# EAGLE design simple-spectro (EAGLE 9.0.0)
DELETE: MF
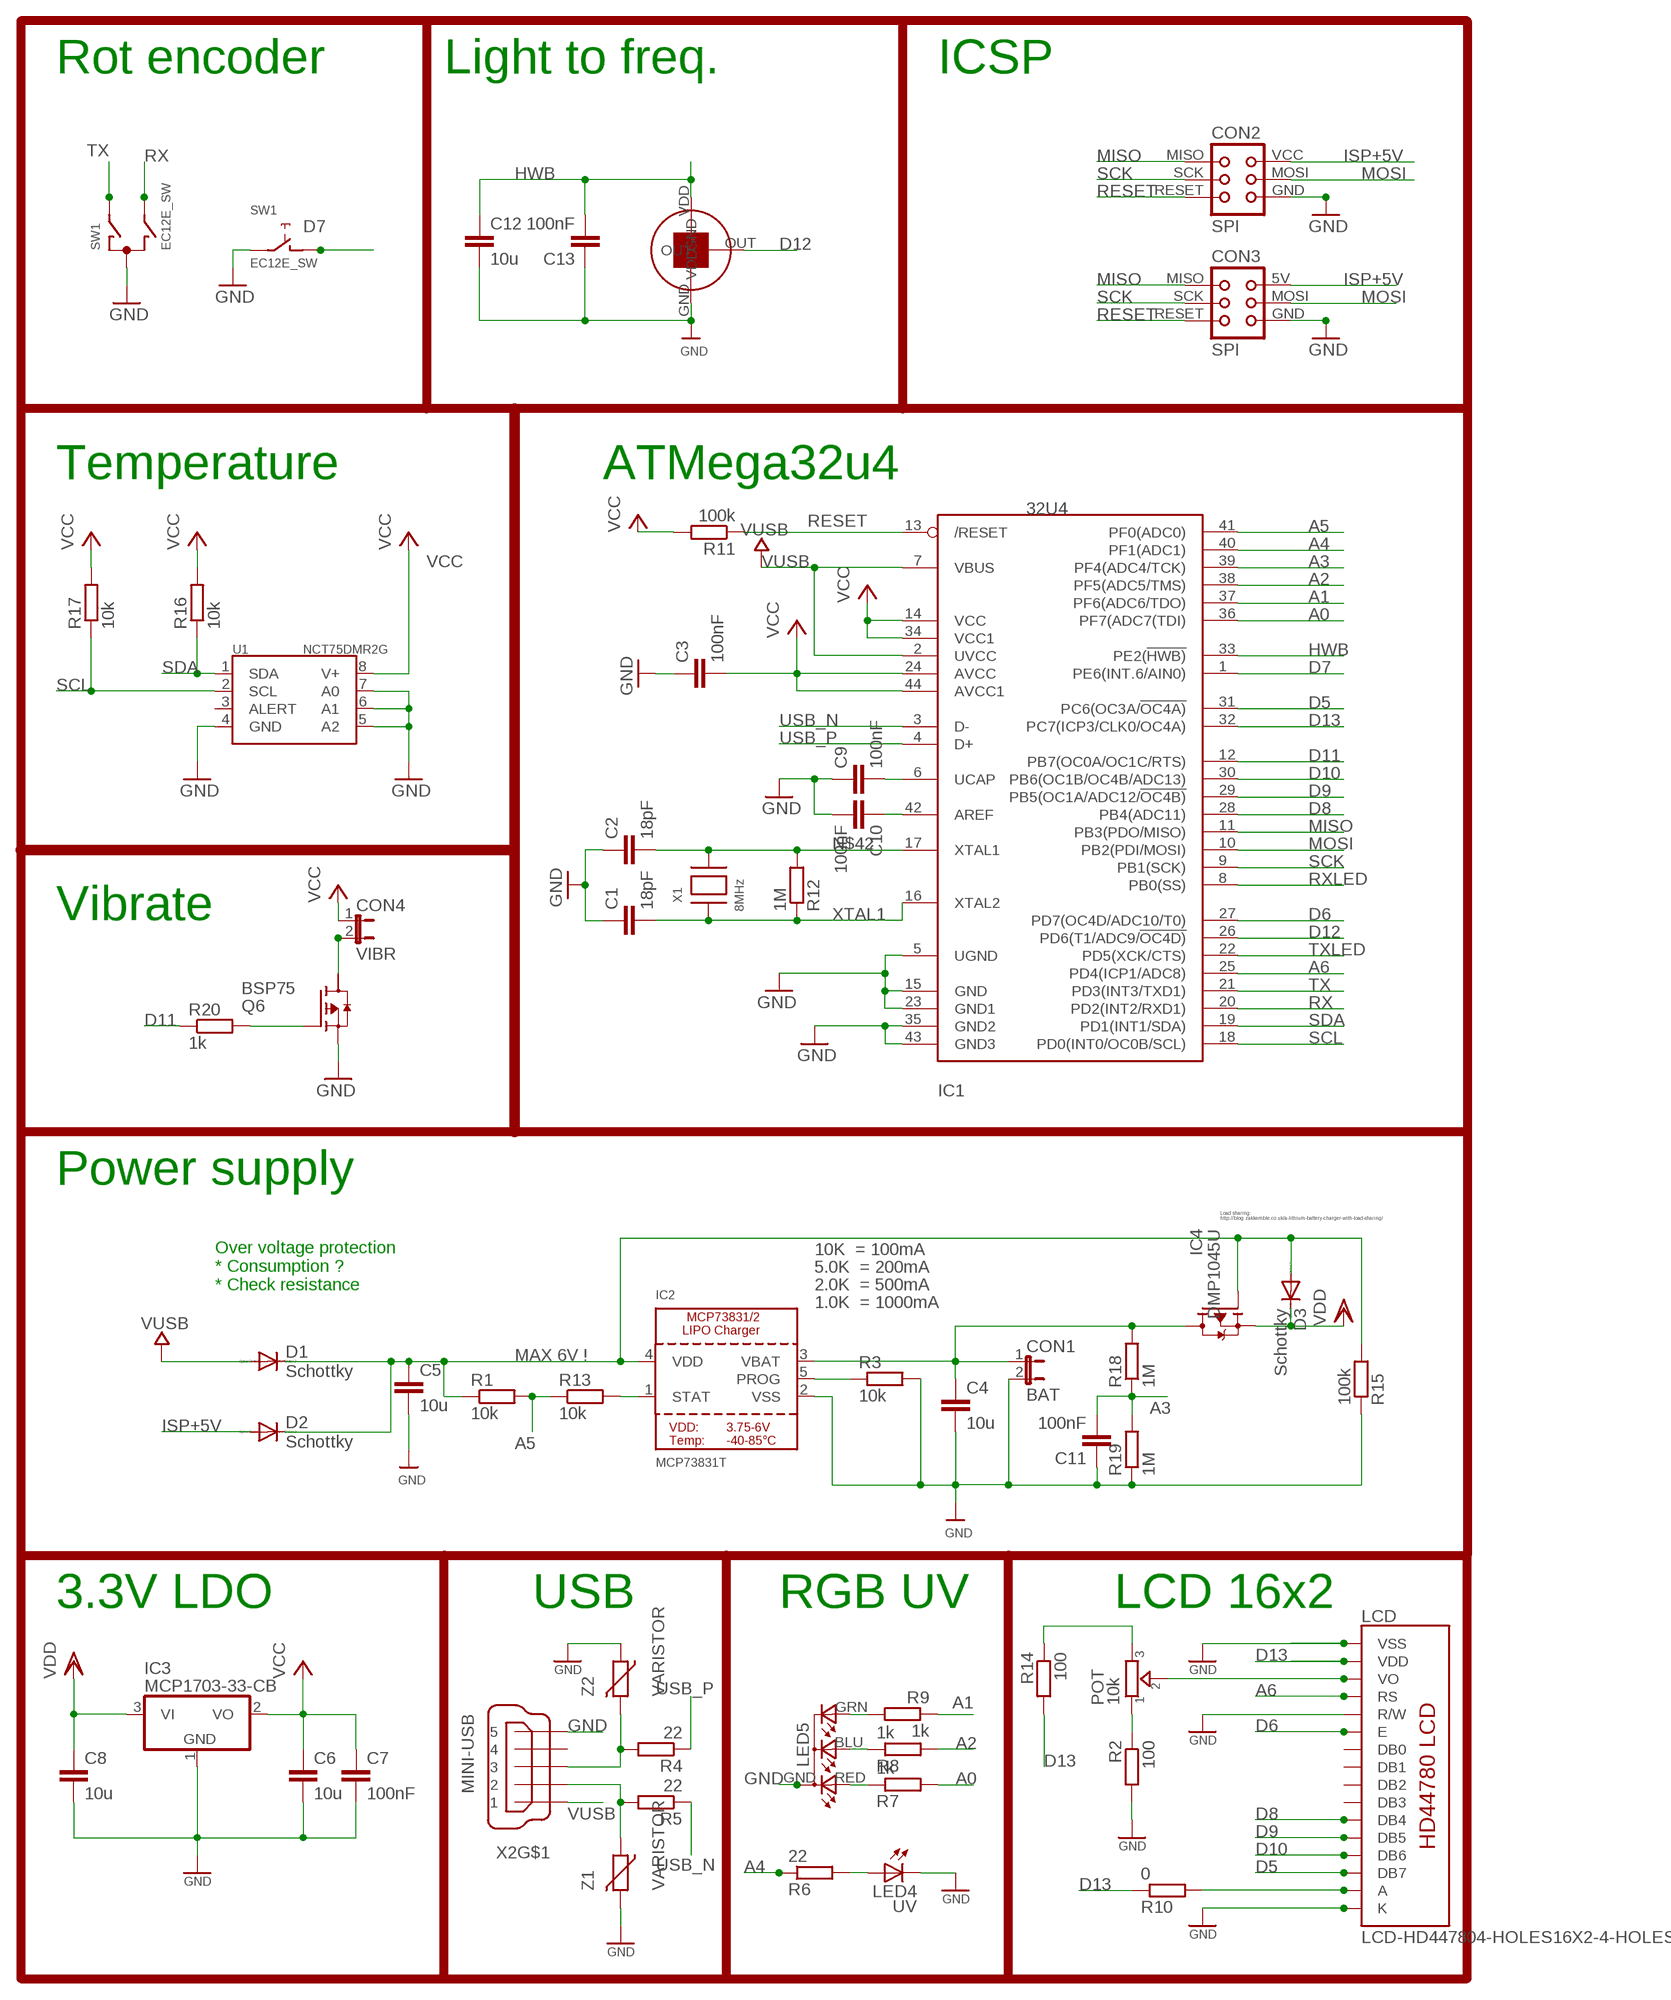
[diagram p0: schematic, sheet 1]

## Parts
C1  18pF  C-EUC0805K  [C0805K]
C2  18pF  C-EUC0805K  [C0805K]
C3  100nF  C-EUC0805K  [C0805K]
C4  10u  C-EUC0805K  [C0805K]
C5  10u  C-EUC0805K  [C0805K]
C6  10u  C-EUC0805K  [C0805K]
C7  100nF  C-EUC0805K  [C0805K]
C8  10u  C-EUC0805K  [C0805K]
C9  100nF  C-EUC0805K  [C0805K]
C10  100nF  C-EUC0805K  [C0805K]
C11  100nF  C-EUC0805K  [C0805K]
C12  10u  C-EUC0805K  [C0805K]
C13  100nF  C-EUC0805K  [C0805K]
CON1  BAT  JP1E  [JP1]
CON2  SPI  TINYISP  [TINYISP]
CON3  SPI  TINYISPT  [TC2030-MCP-NL]
CON4  VIBR  JP1E  [JP1]
D1  Schottky  MBR0520LT  [SOD123]
D2  Schottky  MBR0520LT  [SOD123]
D3  Schottky  MBR0520LT  [SOD123]
IC1  32U4  ATMEGA32U4-AU  [TQFP44]
IC2  MCP73831T  MCP73831/2  [SOT23-5]
IC3  MCP1703-33-CB  MCP1703CB  [SOT23]
IC4  DMP1045U  TRANSISTOR_FET_TSM2301CX  [SOT-23]
LCD  LCD-HD447804-HOLES16X2-4-HOLES  [LCD-16X2-4HOLES]
LED4  UV  LED5MM  [LED5MM]
LED5  RGB-COMMON-CATHODE  [LED-TRICOLOR-THROUGHHOLE]
POT  10k  TRIMMER-3362P  [TRIMMER_3362P]
Q6  BSP75  [PG-SOT-223]
R1  10k  R-EU_R0805  [R0805]
R2  100  R-EU_R0805  [R0805]
R3  10k  R-EU_R0805  [R0805]
R4  22  R-EU_R0805  [R0805]
R5  22  R-EU_R0805  [R0805]
R6  22  R-EU_R0805  [R0805]
R7  1k  R-EU_R0805  [R0805]
R8  1k  R-EU_R0805  [R0805]
R9  1k  R-EU_R0805  [R0805]
R10  0  R-EU_R0805  [R0805]
R11  100k  R-EU_R0805  [R0805]
R12  1M  R-EU_R0805  [R0805]
R13  10k  R-EU_R0805  [R0805]
R14  100  R-EU_R0805  [R0805]
R15  100k  R-EU_R0805  [R0805]
R16  10k  R-EU_R0805  [R0805]
R17  10k  R-EU_R0805  [R0805]
R18  1M  R-EU_R0805  [R0805]
R19  1M  R-EU_R0805  [R0805]
R20  1k  R-EU_R0805  [R0805]
SW1  EC12E_SW  [ALPS_EC12E_SW]
U1  NCT75DMR2G  TMP75DGK  [MSOP8]
U$7  TSL237  [TSL237]
X1  8MHz  XTALNX6035  [NX6035]
X2  MINI-USB  MINI-USB-SCHIELD-32005-201  [32005-201]
Z1  VARISTOR  VARISTORCN0603  [CT/CN0603]
Z2  VARISTOR  VARISTORCN0603  [CT/CN0603]

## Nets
A0: IC1.36(PF7(ADC7(TDI)) R7.2
A1: IC1.37(PF6(ADC6/TDO)) R9.1
A2: IC1.38(PF5(ADC5/TMS)) R8.2
A3: C11.2 IC1.39(PF4(ADC4/TCK)) R18.1 R19.2
A4: IC1.40(PF1(ADC1)) R6.1
A5: IC1.41(PF0(ADC0)) R1.2 R13.1
A6: IC1.25(PD4(ICP1/ADC8)) LCD.4(RS)
AREF: C10.1 IC1.42(AREF)
D5: IC1.31(PC6(OC3A/!OC4A)) LCD.14(DB7)
D6: IC1.27(PD7(OC4D/ADC10/T0)) LCD.6(E)
D7: IC1.1(PE6(INT.6/AIN0)) SW1.D
D8: IC1.28(PB4(ADC11)) LCD.11(DB4)
D9: IC1.29(PB5(OC1A/ADC12/!OC4B)) LCD.12(DB5)
D10: IC1.30(PB6(OC1B/OC4B/ADC13)) LCD.13(DB6)
D11: IC1.12(PB7(OC0A/OC1C/RTS)) R20.1
D12: IC1.26(PD6(T1/ADC9/!OC4D)) U$7.OUT
D13: IC1.32(PC7(ICP3/CLK0/OC4A)) LCD.2(VDD) R10.1 R14.2
GND [power]: C1.1 C2.1 C3.1 C4.2 C5.2 C6.2 C7.2 C8.2 C9.1 C10.2 C11.1 C12.2 C13.1 CON1.2 CON2.GND CON3.GND IC1.5(UGND) IC1.15(GND) IC1.23(GND1) IC1.35(GND2) IC1.43(GND3) IC2.2(VSS) IC3.1(GND) LCD.1(VSS) LCD.5(R/W) LCD.16(K) LED4.K(C) LED5.GND(A2) Q6.3(S) R2.2 R3.2 R15.1 R19.1 SW1.C SW1.E U1.4(GND) U1.5(A2) U1.6(A1) U1.7(A0) U$7.GND X2.5 Z1.2 Z2.1
HWB: C12.1 C13.2 IC1.33(PE2(!HWB)) U$7.VDD
ISP+5V: CON2.VCC CON3.5V(VCC) D2.A
MISO: CON2.MISO CON3.MISO IC1.11(PB3(PDO/MISO))
MOSI: CON2.MOSI CON3.MOSI IC1.10(PB2(PDI/MOSI))
N$1: C9.2 IC1.6(UCAP)
N$2: LCD.3(VO) POT.2
N$3: LED4.A R6.2
N$4: POT.1 R2.1
N$5: IC2.1(STAT) R13.2
N$6: IC2.5(PROG) R3.1
N$8: Q6.1(G) R20.2
N$9: LED5.GRN(CGREEN) R9.2
N$10: LED5.BLU(CBLUE) R8.1
N$11: LCD.15(A) R10.2
N$12: POT.3 R14.1
N$13: LED5.RED(CRED) R7.1
N$14: CON4.2 Q6.2(D)
N$15: C5.1 D1.C D2.C D3.A IC2.4(VDD) IC4.1(G) R1.1 R15.2
N$42: C2.2 IC1.17(XTAL1) R12.2 X1.P$2
RESET: CON2.RESET CON3.RESET IC1.13(/RESET) R11.1
RX: IC1.20(PD2(INT2/RXD1)) SW1.B
RXLED: IC1.8(PB0(SS))
SCK: CON2.SCK CON3.SCK IC1.9(PB1(SCK))
SCL: IC1.18(PD0(INT0/OC0B/SCL)) R17.1 U1.2(SCL)
SDA: IC1.19(PD1(INT1/SDA)) R16.1 U1.1(SDA)
TX: IC1.21(PD3(INT3/TXD1)) SW1.A
TXLED: IC1.22(PD5(XCK/CTS))
USB_N: IC1.3(D-) R5.1
USB_P: IC1.4(D+) R4.1
USBC_N: R5.2 X2.2 Z1.1
USBC_P: R4.2 X2.3 Z2.2
VBAT1: C4.1 CON1.1 IC2.3(VBAT) IC4.3(D) R18.2
VCC: C3.2 C6.1 C7.1 CON4.1 IC1.14(VCC) IC1.24(AVCC) IC1.34(VCC1) IC1.44(AVCC1) IC3.2(VO) R11.2 R16.2 R17.2 U1.8(V+)
VDD [power]: C8.1 D3.C IC3.3(VI) IC4.2(S)
VUSB: D1.A IC1.2(UVCC) IC1.7(VBUS) X2.1
XTAL1: C1.2 IC1.16(XTAL2) R12.1 X1.P$1
Unconnected: LCD.7(DB0) LCD.8(DB1) LCD.9(DB2) LCD.10(DB3) Q6.4(D) SW1.GND1(G) SW1.GND2(G) U1.3(ALERT) X2.4 X2.M1(S:S1) X2.M2(S:S2) X2.M3(S:S3) X2.M4(S:S4)

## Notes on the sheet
- Rot encoder | Light to freq. | ICSP
- Temperature | ATMega32u4
- Vibrate
- Power supply
- Load sharing:
  http://blog.zakkemble.co.uk/a-lithium-battery-charger-with-load-sharing/
- 10K  = 100mA
- 5.0K  = 200mA
- Over voltage protection
  * Consumption ?
  * Check resistance
- 2.0K  = 500mA
- 1.0K  = 1000mA
- MAX 6V !
- 3.3V LDO | USB | RGB UV | LCD 16x2

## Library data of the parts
C1 C2 = rcl:C-EU: CAPACITOR, European symbol; ELECROW: C1797; LCSC: C1797; MPN: 77-VJ1206A180JXXPBC
C3 C7 C9-C11 C13 = rcl:C-EU: CAPACITOR, European symbol; ELECROW: C49678; LCSC: C49678; MPN: 80-C1206C104K5R
C4-C6 C8 C12 = rcl:C-EU: CAPACITOR, European symbol; ELECROW: C15850; LCSC: C15850; MPN: 77-VJ1206V106ZXQTBC
CON1 CON4 = jumper:JP1E: JUMPER
CON2 = lpatiny:TINYISP: CONNECTOR; OC_FARNELL: unknown; OC_NEWARK: unknown
CON3 = lpatiny:TINYISP: CONNECTOR
D1-D3 = diode:MBR0520LT: SCHOTTKY BARRIER RECTIFIER; LCSC: C82544; MPN: 621-1N5819HW-F
IC1 = adafruit:ATMEGA32U4: http://www.ladyada.net/library/eagle; LCSC: C44854; MPN: 556-ATMEGA32U4RC-AU
IC2 = microbuilder:MCP73831/2: MCP73831/2 LIPO Charger VDD: 3.75 - 6V Temp -40 - 85°C Programmable Charge Rate: 15-500mA NOTE: STAT is a tri-state logic output on the MCP73831 and an open-drain output on the MCP73832. SOT23-5 with 4.2V output and tri-state logic on STAT = MCP73831T-2ACI/OT; LCSC: C14879; MPN: 579-MCP73831T-3ACIOT
IC3 = linear:MCP1703: 250 mA, 16V, Low Quiescent Current LDO Regulator Source: http://ww1.microchip.com/downloads/en/DeviceDoc/22049b.pdf; LCSC: C53352
IC4 = dp_devices:TRANSISTOR_FET_TSM2301CX: 20V P-Channel Enhancement Mode MOSFET; LCSC: C110499; MPN: 621-DMP1045U-7
LCD = HD44780LCD:LCD-HD44780
LED4 = SparkFun:LED: LEDs
LED5 = lpatiny:RGB-COMMON-CATHODE
POT = dp_devices:TRIMMER: Trimmer resistor
Q6 = lpatiny:BSP75: SIPMOS (R) Small-Signal-Transistor P-Channel (2 Drain) Source: http://www.infineon.com/dgdl/BSP613P_Rev2.4.pdf; OC_FARNELL: unknown; OC_NEWARK: unknown
R1 R3 R13 R16 R17 = rcl:R-EU_: RESISTOR, European symbol; ELECROW: C17414; LCSC: C17414
R2 R14 = rcl:R-EU_: RESISTOR, European symbol; ELECROW: C17408; LCSC: C17408
R4 R5 = rcl:R-EU_: RESISTOR, European symbol; ELECROW: C17561; LCSC: C17561
R6 = rcl:R-EU_: RESISTOR, European symbol; ELECROW: C17561; LCSC: C17561; MPN: 667-ERJ-8GEYJ101V
R7-R9 R20 = rcl:R-EU_: RESISTOR, European symbol; ELECROW: C17513; LCSC: C17513
R10 = rcl:R-EU_: RESISTOR, European symbol; ELECROW: C17477; LCSC: C17477
R11 R15 = rcl:R-EU_: RESISTOR, European symbol; ELECROW: C17407; LCSC: C17407; MPN: RC1206FR-07100KL
R12 R18 R19 = rcl:R-EU_: RESISTOR, European symbol; ELECROW: C17514; LCSC: C17514
SW1 = switch-alps:EC12E_SW: ALPS rotary Encoder EC12E series with switch; MPN: EC12E2424407; OC_FARNELL: 1520813; OC_NEWARK: 74M1068
U1 = ti_tmp:TMP75; LCSC: C94387
U$7 = lpatiny:TSL237
X1 = lpatiny:XTAL: Low cost SMT crystals, no capacitors included; LCSC: C122522; MPN: 729-F60800010
X2 = con-cypressindustries:MINI-USB-SCHIELD-: MINI USB-B Conector Source: www.cypressindustries.com; LCSC: C46391; MPN: 649-10033526-N3212LF
Z1 Z2 = varistor:VARISTOR: VARISTOR; LCSC: C126845

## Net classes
0 default: width 0.406 mm, clearance 0.25 mm
1 power: width 0.406 mm, drill 0.305 mm, clearance 0.25 mm
2 VIN: width 0.406 mm, clearance 0.25 mm
3 fine: width 0.406 mm, clearance 0.25 mm
4 aref: width 0.406 mm, clearance 0.25 mm

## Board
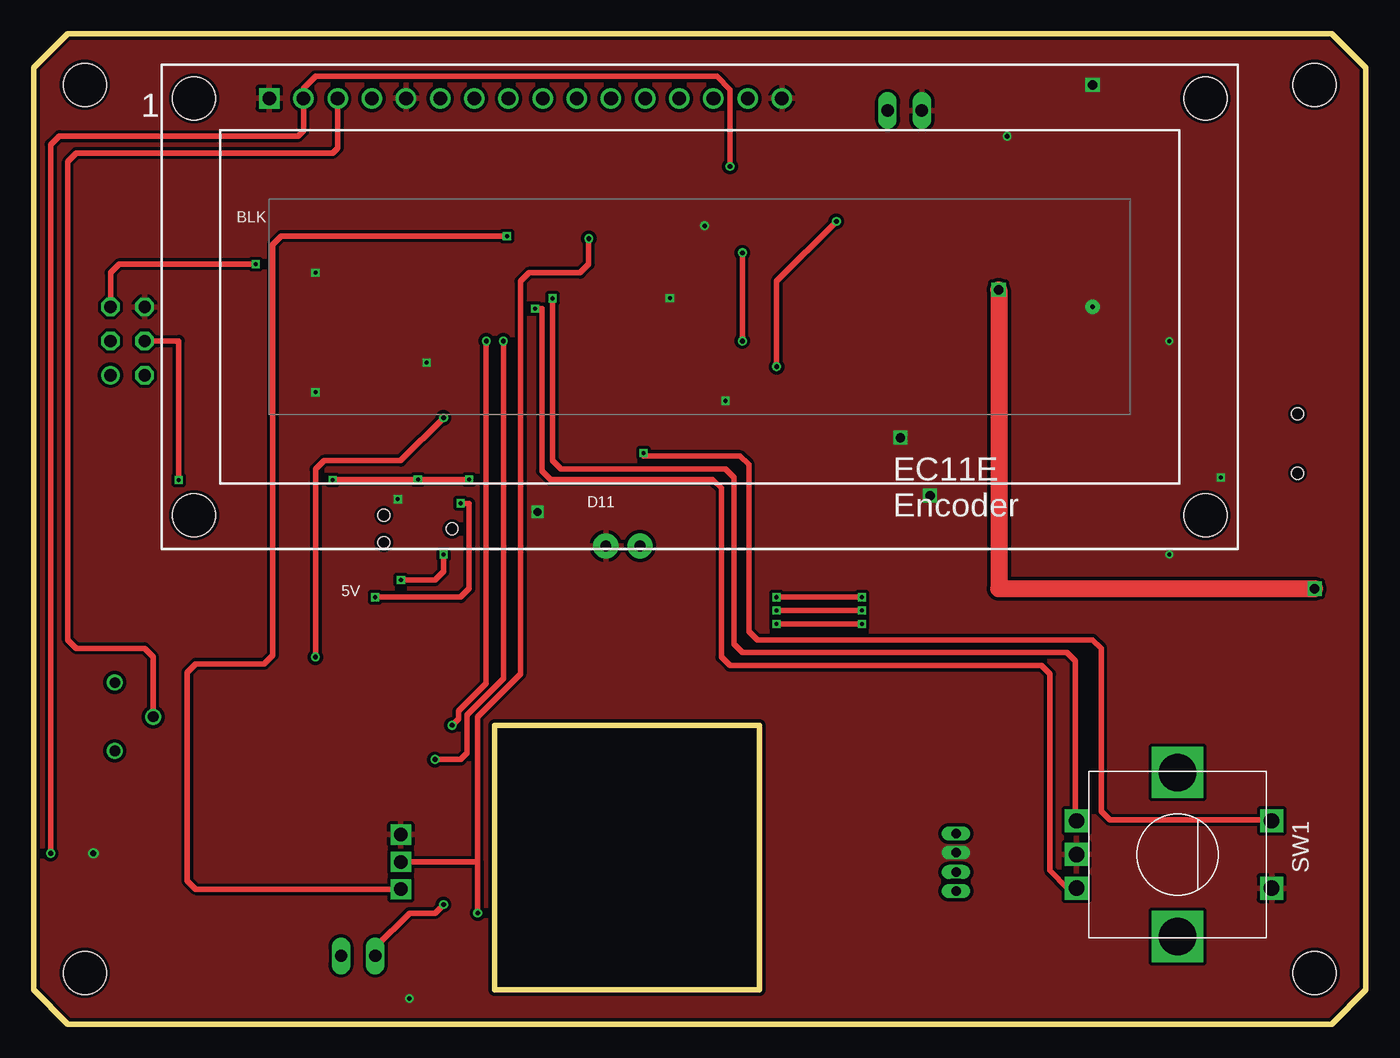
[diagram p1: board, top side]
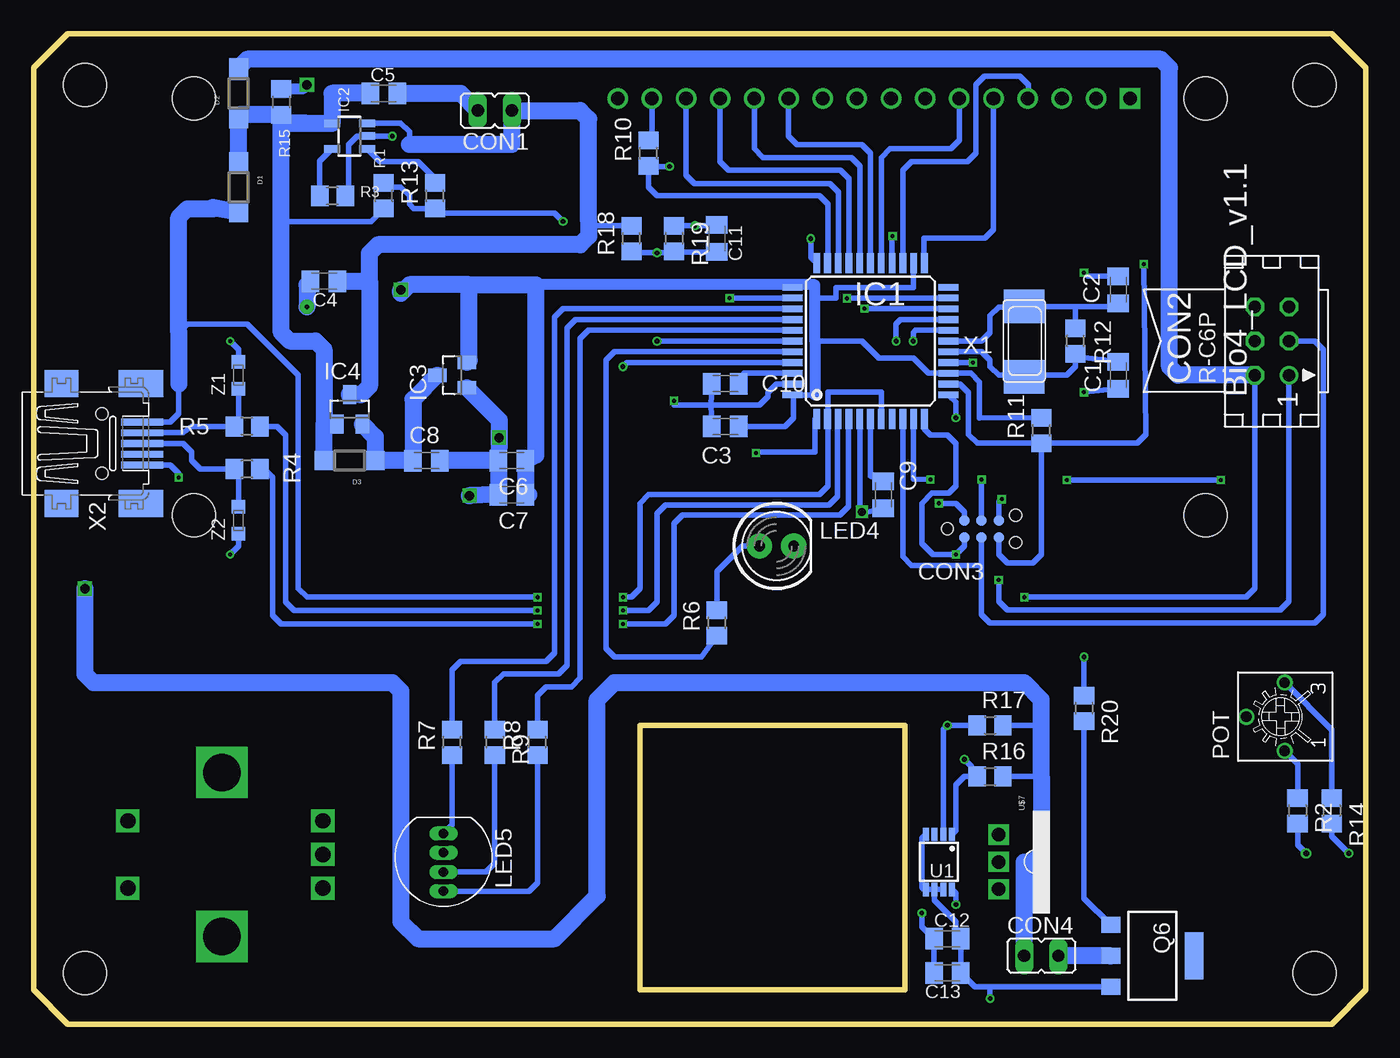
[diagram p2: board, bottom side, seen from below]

Size 99.06 x 73.66 mm. Coordinates in mm from the lower left corner, seen from the top.
Outline: 34.29,22.23 53.98,22.23 53.98,2.54 34.29,2.54 34.29,22.23
Outline: 0,71.12 0,2.54 2.54,0 96.52,0 99.06,2.54 99.06,71.12 96.52,73.66 2.54,73.66 0,71.12
Copper layers (1*16): Top 0.035mm / dielectric 0.2mm / Bottom 0.035mm
Design rules "SeeedStudio_DRU_no_angle_20130527 *": minimum track width 6mil, minimum drill 12mil, track to track 6mil, track to pad 6mil, pad to pad 6mil, via to via 6mil, smd to smd 0mil, copper to edge 10mil, drill to drill 10mil, minimum pad ring 6mil, minimum via ring 6mil, stop-mask expansion 2mil, vias tented up to drill 25mil, thermal gap 10mil
Holes 3.2 mm at 3.81,69.85 3.81,3.81 95.25,69.85 95.25,3.81

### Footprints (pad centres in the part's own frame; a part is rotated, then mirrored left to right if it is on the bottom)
C0805K = smd 1.3 x 1.6: 1 -1,0; 2 1,0
JP1 = drill 0.914 long: 1 0,-1.27; 2 0,1.27
TINYISP = drill 0.914 octagon: GND 2.54,1.27; MOSI 0,1.27; RESET 2.54,-1.27; SCK 0,-1.27; VCC -2.54,1.27 | drill 0.914: MISO -2.54,-1.27
TC2030-MCP-NL = smd 0.787 x 0.787: 5V 1.27,0.635; GND 3.81,0.635; MISO 1.27,-0.635; MOSI 2.54,0.635; RESET 3.81,-0.635; SCK 2.54,-0.635 | hole 0.889: 0,0; 5.08,-1.016; 5.08,1.016
SOD123 = smd 1.4 x 1.4: A 1.9,0; C -1.9,0
TQFP44 = smd 1.5 x 0.5: 1 -5.8,4; 2 -5.8,3.2; 3 -5.8,2.4; 4 -5.8,1.6; 5 -5.8,0.8; 6 -5.8,0; 7 -5.8,-0.8; 8 -5.8,-1.6; 9 -5.8,-2.4; 10 -5.8,-3.2; 11 -5.8,-4; 23 5.8,-4; 24 5.8,-3.2; 25 5.8,-2.4; 26 5.8,-1.6; 27 5.8,-0.8; 28 5.8,0; 29 5.8,0.8; 30 5.8,1.6; 31 5.8,2.4; 32 5.8,3.2; 33 5.8,4 | smd 0.5 x 1.5: 12 -4,-5.8; 13 -3.2,-5.8; 14 -2.4,-5.8; 15 -1.6,-5.8; 16 -0.8,-5.8; 17 0,-5.8; 18 0.8,-5.8; 19 1.6,-5.8; 20 2.4,-5.8; 21 3.2,-5.8; 22 4,-5.8; 34 4,5.8; 35 3.2,5.8; 36 2.4,5.8; 37 1.6,5.8; 38 0.8,5.8; 39 0,5.8; 40 -0.8,5.8; 41 -1.6,5.8; 42 -2.4,5.8; 43 -3.2,5.8; 44 -4,5.8
SOT23-5 = smd 0.55 x 1.2: 1 -0.95,-1.3; 2 0,-1.3; 3 0.95,-1.3; 4 0.95,1.3; 5 -0.95,1.3
SOT23 = smd 1 x 1.4: 1 -0.95,-1.1; 2 0.95,-1.1; 3 0,1.1
SOT-23 = smd 1 x 1.4: 1 -0.95,-1.1; 2 0.95,-1.1; 3 0,1.1
LCD-16X2-4HOLES = drill 1.016 square: 1 -32,15.5 | drill 1.016: 2 -29.46,15.5; 3 -26.92,15.5; 4 -24.38,15.5; 5 -21.84,15.5; 6 -19.3,15.5; 7 -16.76,15.5; 8 -14.22,15.5; 9 -11.68,15.5; 10 -9.14,15.5; 11 -6.6,15.5; 12 -4.06,15.5; 13 -1.52,15.5; 14 1.02,15.5; 15 3.56,15.5; 16 6.1,15.5 | hole 3.2: -37.6,15.5; -37.6,-15.5; 37.6,-15.5; 37.6,15.5
LED5MM = drill 0.813 pad 1.88: A -1.27,0; K 1.27,0
LED-TRICOLOR-THROUGHHOLE = drill 0.7 long: BLU 2.175,0; GND -0.682,0; GRN 0.746,0; RED -2.111,0
TRIMMER_3362P = drill 0.8: 1 -2.54,-0.31; 2 0,2.54; 3 2.54,-0.31
PG-SOT-223 = smd 1.2 x 1.4: 1 -2.311,-3.099; 2 0,-3.099; 3 2.311,-3.099 | smd 3.5 x 1.4: 4 0,3.099
R0805 = smd 1.3 x 1.5: 1 -0.95,0; 2 0.95,0
ALPS_EC12E_SW = drill 1.143 square: A -2.5,-7.5; B 2.5,-7.5; C 0,-7.5; D -2.5,7; E 2.5,7 | drill 2.794 square: GND1 -6.1,0; GND2 6.1,0
MSOP8 = smd 0.45 x 1: 1 -0.975,-2.05; 2 -0.325,-2.05; 3 0.325,-2.05; 4 0.975,-2.05; 5 0.975,2.05; 6 0.325,2.05; 7 -0.325,2.05; 8 -0.975,2.05
TSL237 = drill 1 pad 1.27 square: GND -2.032,-2.54; OUT 2.032,-2.54; VDD 0,-2.54
NX6035 = smd 2.5 x 3: P$1 2.665,0; P$2 -2.565,0
32005-201 = smd 3.1 x 0.5: 1 3,1.6; 2 3,0.8; 3 3,0; 4 3,-0.8; 5 3,-1.6 | smd 2.5 x 2: M1 -3,-4.45; M2 -3,4.45 | smd 3.3 x 2: M3 2.9,4.45; M4 2.9,-4.45 | hole 0.9: 0,2.2; 0,-2.2
CT/CN0603 = smd 1 x 1: 1 -1,0; 2 1,0

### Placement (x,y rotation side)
C1  18.41,48.26 90 bottom
C2  18.41,54.61 270 bottom
C3  47.62,44.45 0 bottom
C4  77.47,55.24 180 bottom
C5  73.03,69.22 0 bottom
C6  63.5,41.91 180 bottom
C7  63.5,39.37 180 bottom
C8  69.85,41.91 0 bottom
C9  35.88,39.37 90 bottom
C10  47.62,47.62 180 bottom
C11  48.26,58.42 270 bottom
C12  31.11,6.35 0 bottom
C13  31.11,3.81 180 bottom
CON1  64.77,67.94 90 bottom
CON2  6.99,50.8 90 bottom
CON3  31.11,36.83 0 bottom
CON4  24.13,5.08 270 bottom
D1  83.82,62.23 270 bottom
D2  83.82,69.22 90 bottom
D3  75.56,41.91 180 bottom
IC1  36.83,50.8 90 bottom
IC2  75.56,66.04 90 bottom
IC3  67.94,48.26 90 bottom
IC4  75.56,45.72 0 bottom
LCD  49.53,53.34 0 top
LED4  43.81,35.56 0 bottom
LED5  68.58,12.06 270 bottom
POT  6.35,22.86 90 bottom
Q6  15.88,5.08 270 bottom
R1  73.03,61.59 90 bottom
R2  5.08,15.88 270 bottom
R3  76.83,61.59 0 bottom
R4  83.19,41.27 180 bottom
R5  83.19,44.45 180 bottom
R6  48.26,29.84 90 bottom
R7  67.94,20.95 90 bottom
R8  61.59,20.95 90 bottom
R9  64.77,20.95 270 bottom
R10  53.34,64.77 90 bottom
R11  24.13,44.16 90 bottom
R12  21.59,50.8 90 bottom
R13  69.22,61.59 90 bottom
R14  2.54,15.88 270 bottom
R15  80.64,68.58 270 bottom
R16  27.94,18.41 0 bottom
R17  27.94,22.23 0 bottom
R18  54.61,58.42 90 bottom
R19  51.44,58.42 270 bottom
R20  20.95,23.5 270 bottom
SW1  85.05,12.62 270 top
U1  31.75,12.06 180 bottom
U$7  24.77,12.06 270 bottom
X1  25.4,50.8 270 bottom
X2  93.98,43.18 0 bottom
Z1  83.82,48.26 90 bottom
Z2  83.82,37.47 90 bottom

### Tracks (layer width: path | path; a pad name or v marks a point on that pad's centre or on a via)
A0
  Bottom 0.406: IC1.36 59.69,53.2 60.33,52.56 60.33,27.61 60.96,26.98 67.31,26.98 67.94,26.34 R7.2
A1
  Bottom 0.406: IC1.37 58.78,52.4 59.41,51.77 59.41,26.67 60.05,26.04 64.14,26.04 64.77,25.4 R9.1
A2
  Bottom 0.406: IC1.38 57.78,51.6 58.42,50.97 58.42,25.73 59.05,25.09 60.96,25.09 61.59,24.46 R8.2
A3  (via drill 0.35)
  Top 0.406: v52.7,50.8 v52.7,57.36
  Bottom 0.406: IC1.39 v52.7,50.8 | R18.1 54.5,57.36 v52.7,57.36 50.91,57.36 R19.2 51.38,57.42 C11.2
A4
  Bottom 0.406: 42.63,50.04 IC1.40 55.88,50 56.52,49.37 56.52,27.94 55.88,27.3 49.4,27.3 R6.1
A5  (via drill 0.35)
  Top 0.406: v59.69,59.69 55.24,55.24 v55.24,48.9
  Bottom 0.406: 73.19,62.71 R1.2 72.71,62.23 71.75,62.23 71.12,61.59 71.12,60.96 70.81,60.65 R13.1 68.89,60.33 60.33,60.33 v59.69,59.69 | v55.24,48.9 54.94,49.2 52.7,49.2 IC1.41
A6
  Bottom 0.406: LCD.4 25.08,68.84 25.08,69.85 25.72,70.48 28.36,70.48 29,69.85 29,64.77 29.64,64.14 33.8,64.14 34.43,63.5 IC1.25
AREF
  Bottom 0.406: IC1.42 46.23,48.4 C10.1
D5
  Bottom 0.406: 39.24,56.6 IC1.31 39.23,61.87 39.87,62.5 49.91,62.5 50.55,63.14 LCD.14
D6
  Bottom 0.406: IC1.27 36.03,64.45 35.4,65.09 30.86,65.09 30.23,65.72 LCD.6
D7  (via drill 0.3)
  Top 0.406: v45.34,42.48 45.34,42.24 52.54,42.24 53.17,41.6 53.17,29.21 53.81,28.57 78.74,28.57 79.38,27.94 79.38,15.84 80.01,15.2 91.97,15.2 SW1.D
  Bottom 0.406: IC1.1 40.96,45 40.96,42.55 45.34,42.55 v45.34,42.48
D8
  Bottom 0.406: LCD.11 42.93,66.04 42.3,65.41 37.47,65.41 36.83,64.77 IC1.28
D9
  Bottom 0.406: LCD.12 45.47,65.09 44.84,64.45 38.27,64.45 37.63,63.82 IC1.29
D10
  Bottom 0.406: LCD.13 48.01,64.14 47.38,63.5 39.06,63.5 38.43,62.87 IC1.30
D11  (via drill 0.35)
  Top 0.406: v30.48,45.09 27.3,41.91 21.59,41.91 20.95,41.27 v20.95,27.3
  Bottom 0.406: IC1.12 30.48,46.25 v30.48,45.09 | v20.95,27.3 R20.1
D12  (via drill 0.3)
  Top 0.406: v35.19,58.61 18.41,58.61 17.78,57.98 17.78,27.43 17.14,26.8 12.06,26.8 11.43,26.16 11.43,10.67 12.06,10.03 U$7.OUT
  Bottom 0.406: IC1.26 35.24,58.51 35.19,58.51 v35.19,58.61
D13  (via drill 0.35)
  Top 0.406: v51.78,63.78 51.78,69.51 50.8,70.48 20.95,70.48 20.07,69.6 LCD.2 20.07,66.42 19.68,66.04 1.91,66.04 1.27,65.41 v1.27,12.7
  Bottom 0.406: IC1.32 40.01,56.6 40.01,60.96 40.64,61.59 52.7,61.59 53.34,62.23 R10.1 53.3,63.78 v51.78,63.78 | v1.27,12.7 2.54,13.97 R14.2
GND  (via drill 0.3, 0.35, 0.35 pad 1.05, 0.45, 0.6, 0.7)
  Bottom 0.406: 49.02,47.6 C10.2 48.68,46.04 | 48.68,46.04 C3.1 | IC1.43 43.81,47.6 44.45,46.97 44.45,46.67 45.09,46.04 48.68,46.04 | v51.44,46.35 51.44,46.04 48.68,46.04 | C9.1 37.47,37.97 | IC1.5 37.63,37.97 37.47,37.97 | LCD.5 27.69,59.08 28.32,58.45 32.85,58.45 32.85,56.6 IC1.23 | 64.77,41.91 C6.2 | C7.2 64.77,39.37 | X2.5 88.9,41.58 88.27,40.95 v88.27,40.64 | IC1.35 v47.3,54 | IC1.15 v29.22,49.2 | v29.22,49.2 | CON3.GND 27.3,38.81 v27.08,39.04 | 37.47,37.97 v37.47,38.1 | C1.1 v20.95,46.99 | 76.2,61.59 R3.2 75.65,61.59 75.65,65.41 75.01,66.04 IC2.2 v72.39,66.04 | U1.7 U1.6 | U1.6 U1.5 32.88,10.02 33.02,10.16 33.02,13.82 U1.4 | v20.95,55.88 20.68,55.61 C2.1 | R19.1 v49.89,59.37 48.31,59.37 C11.1 | R2.2 5.08,13.34 v4.45,12.7 | 27.94,2.77 Q6.3 | U1.6 32.08,9.21 30.48,7.62 30.48,6.71 C12.2 C13.1 29.07,2.77 27.94,2.77 | v27.94,1.91 27.94,2.77 | Z1.2 83.82,50.16 v84.45,50.8 | Z2.1 83.82,35.56 v84.45,34.92
  Bottom 0.813: v78.74,69.85 79.06,69.53 R15.1
  Bottom 1.27: C6.2 v64.45,43.62 64.45,44.91 IC3.1 | C6.2 C8.2 | C6.2 C7.2 | 64.77,39.37 v66.66,39.3 | C5.2 67.31,69.22 CON1.2 | C4.2 78.74,54.98 v78.74,53.34
  pour Top: 0,71.12 0,2.54 2.54,0 96.52,0 99.06,2.54 99.06,71.12 96.52,73.66 2.54,73.66
HWB  (via drill 0.35)
  Top 0.406: v41.27,58.42 41.27,56.52 40.64,55.88 36.83,55.88 36.2,55.24 36.2,26.04 33.02,22.86 33.02,12.06 | 33.02,12.06 v33.02,8.26 | U$7.VDD 33.02,12.06
  Bottom 0.406: 40.83,56.7 IC1.33 41.27,57.05 v41.27,58.42 | C13.2 C12.1 33.02,7.25 v33.02,8.26
ISP+5V  (via drill 0.3)
  Top 0.406: v31.75,38.73 32.38,38.73 32.38,32.38 31.75,31.75 v25.4,31.75
  Bottom 0.406: CON3.5V 29.84,38.1 30.48,38.73 v31.75,38.73 | v25.4,31.75 8.89,31.75 8.26,32.38 CON2.VCC
  Bottom 1.27: CON2.VCC 13.97,48.26 14.61,48.9 14.61,71.12 15.24,71.75 83.19,71.75 D2.A
MISO  (via drill 0.3)
  Top 0.406: v27.3,33.02 29.84,33.02 30.48,33.66 v30.48,34.92
  Bottom 0.406: CON3.MISO 29.84,35.56 v30.48,34.92 32.2,34.92 33.02,35.75 33.02,38.73 32.26,39.49 30.99,39.49 30.48,40.01 30.48,43.18 31.11,43.81 32.38,43.81 32.83,44.26 IC1.11 | CON2.MISO 5.71,31.42 6.35,30.79 26.67,30.79 27.3,31.42 v27.3,33.02
MOSI  (via drill 0.3)
  Top 0.406: v32.38,40.5 v28.57,40.5 22.23,40.5 v22.23,40.47 | CON2.MOSI 10.79,50.8 v10.79,40.47
  Bottom 0.406: CON3.MOSI v28.57,40.5 | v22.23,40.47 v10.79,40.47 | IC1.10 33.63,40.52 v32.38,40.5
N$1
  Bottom 0.406: C9.2 36.83,40.77 IC1.6
N$2
  Top 0.406: LCD.3 22.61,65.16 22.23,64.77 3.17,64.77 2.54,64.14 2.54,28.57 3.17,27.94 8.26,27.94 8.89,27.3 POT.2
  Bottom 0.406: LCD.3
N$3
  Bottom 0.406: R6.2 48.26,33.66 46.35,35.56 LED4.A
N$4
  Bottom 0.406: R2.1 5.08,19.36 POT.1
N$5
  Bottom 0.406: IC2.1 73.31,64.14 70.48,64.14 69.22,62.87 R13.2
N$6
  Bottom 0.406: IC2.5 77.78,64.17 R3.1
N$8
  Bottom 0.406: Q6.1 20.95,9.37 R20.2
N$9
  Bottom 0.406: LED5.GRN 65.41,11.32 64.77,11.95 R9.2
N$10
  Bottom 0.406: LED5.BLU 62.23,9.89 61.59,10.53 R8.1
N$11
  Bottom 0.406: LCD.15 53.09,66.42 R10.2
N$12
  Bottom 0.406: R14.1 2.54,21.9 POT.3
N$13
  Bottom 0.406: R7.1 67.94,14.81 LED5.RED
N$14
  Bottom 1.27: Q6.2 CON4.2
N$15
  Bottom 0.406: 77.06,44.62 IC4.1 | 80.64,59.69 73.98,59.69 R1.1
  Bottom 1.27: D1.C D2.C 83.82,67.63 R15.2 80.64,66.99 78.76,66.99 | 77.47,44.62 77.06,44.62 | 77.47,44.62 77.47,50.16 78.11,50.8 80.01,50.8 80.64,51.44 80.64,59.69 80.64,66.97 78.76,66.99 | 78.76,66.99 IC2.4 76.86,69.22 C5.1 | D3.A 77.47,44.62
N$42
  Bottom 0.406: IC1.17 28.57,50.8 27.94,51.44 27.94,52.7 27.3,53.34 25.4,53.34 X1.P$2 21.59,53.37 | 21.59,53.37 R12.2 | C2.2 18.66,53.37 21.59,53.37
RESET  (via drill 0.3)
  Top 0.406: v16.51,56.52 6.35,56.52 5.71,55.88 CON2.RESET
  Bottom 0.406: IC1.13 30.18,47.6 29.54,46.97 29.54,43.84 28.9,43.21 R11.1 | CON3.RESET 27.3,34.92 26.67,34.29 24.77,34.29 24.13,34.92 R11.1 | R11.1 16.98,43.21 16.35,43.85 v16.51,56.52
RX  (via drill 0.3)
  Top 0.406: v37.27,53.21 37.8,53.21 37.8,41.13 38.43,40.5 50.49,40.5 51.13,39.87 51.13,27.3 51.77,26.67 74.93,26.67 75.56,26.04 75.56,11.43 76.88,10.12 SW1.B
  Bottom 0.406: IC1.20 34.1,53.2 v37.27,53.21
SCK
  Bottom 0.406: CON3.SCK 28.57,34.12 | 28.57,34.12 33.8,34.12 34.43,34.76 IC1.9 | CON2.SCK 3.81,50.8 3.17,50.16 3.17,30.48 3.81,29.84 27.94,29.84 28.57,30.48 28.57,34.12
SCL  (via drill 0.35)
  Top 0.406: v31.11,22.23 31.58,22.69 31.58,23.28 33.66,25.35 v33.66,50.8
  Bottom 0.406: U1.2 31.43,21.91 v31.11,22.23 R17.1 | IC1.18 33.49,51.6 33.66,51.44 v33.66,50.8
SDA  (via drill 0.35)
  Top 0.406: v29.84,19.68 31.75,19.68 32.24,20.17 32.24,23.01 34.92,25.69 v34.92,50.8
  Bottom 0.406: IC1.19 34.59,52.4 34.92,52.07 v34.92,50.8 | v29.84,19.68 29.34,19.18 R16.1 29.84,18.41 30.48,17.78 30.48,14.41 U1.1
TX  (via drill 0.3)
  Top 0.406: v38.59,53.98 38.59,41.91 39.23,41.27 51.44,41.27 52.07,40.64 52.07,28.27 52.7,27.64 76.83,27.64 77.47,27 77.47,15.2 SW1.A
  Bottom 0.406: IC1.21 v38.59,53.98
USB_N  (via drill 0.3)
  Top 0.406: v55.24,30.76 v61.58,30.76
  Bottom 0.406: IC1.3 39.29,45 39.29,39.25 39.93,38.61 52.07,38.61 52.7,37.98 52.7,31.39 53.34,30.76 v55.24,30.76 | v61.58,30.76 79.69,30.76 80.33,31.39 80.33,43.81 80.96,44.45 R5.1
USB_P  (via drill 0.3)
  Top 0.406: v55.24,29.77 v61.58,29.77
  Bottom 0.406: v61.58,29.77 80.64,29.77 81.28,30.4 81.28,40.64 81.92,41.27 R4.1 | IC1.4 38.47,45 38.47,38.49 39.1,37.86 50.8,37.86 51.44,37.22 51.44,30.4 52.07,29.77 v55.24,29.77
USBC_N
  Bottom 0.406: X2.2 87.94,43.98 87.3,44.45 R5.2 83.82,44.77 Z1.1
USBC_P
  Bottom 0.406: X2.3 87.94,43.18 87.3,42.55 87.3,41.91 86.67,41.27 R4.2 83.82,40.96 Z2.2
VBAT1
  Bottom 0.406: IC2.3 71.75,66.99 71.12,66.36 71.12,65.41 | 57.66,59.82 57.78,59.69 57.47,59.37 R18.2
  Bottom 1.27: 71.12,65.41 63.5,65.41 CON1.1 58.42,67.94 57.78,67.31 57.78,59.69 57.78,58.59 58.42,57.96 73.45,57.96 74.08,57.32 74.08,55.24 | 74.08,55.24 74.08,47.44 74.72,46.81 75.56,46.81 IC4.3 | C4.1 74.08,55.24
VCC  (via drill 0.35, 0.7)
  Top 0.406: v30.48,8.89 29.84,8.26 27.94,8.26 25.4,5.71 CON4.1
  Top 1.27: v71.75,54.61 71.75,32.38 v95.25,32.38
  Bottom 0.406: C3.2 43.18,44.45 42.55,45.09 42.55,46.8 IC1.44 40.98,46.8 40.94,48.27 | R11.2 28.74,45.06 28.74,47.77 29.38,48.4 IC1.14 32.52,48.4 33.66,49.53 36.2,49.53 37.47,50.8 40.98,50.8 | 40.94,48.27 40.8,53.98 | 40.8,53.98 40.8,54.8 IC1.34 | IC1.24 33.66,56.6 33.66,54.77 39.4,54.77 39.4,53.98 40.8,53.98 | R17.2 24.13,22.23 | R16.2 24.13,18.41 | 40.81,48.4 40.94,48.27 | v30.48,8.89 30.48,9.72 U1.8
  Bottom 0.813: 61.72,54.98 40.98,54.98 40.98,50.8 40.98,46.8
  Bottom 1.27: 62.23,39.37 C7.1 C6.1 61.72,42.29 61.72,54.98 66.67,54.98 | 66.67,54.98 71.12,54.98 71.75,54.34 v71.75,54.61 | v95.25,32.38 95.25,26.04 94.61,25.4 72.39,25.4 71.75,24.77 71.75,7.62 70.48,6.35 60.33,6.35 57.15,9.53 57.15,24.13 55.88,25.4 25.4,25.4 24.13,24.13 24.13,22.23 24.13,18.41 24.13,12.7 24.77,12.06 25.4,12.06 CON4.1 | 24.13,45.09 R11.2 | IC3.2 66.67,49.38 66.67,54.98
VDD
  Bottom 1.27: IC4.2 73.67,43.67 D3.C C8.1 70.85,46.45 IC3.3
VUSB  (via drill 0.3)
  Top 0.406: v55.24,31.75 v61.58,31.75
  Bottom 0.406: 40.01,45 40.01,46.99 36.03,46.99 IC1.7 | IC1.2 40.01,45 | 40.01,45 40.01,40.01 40.64,39.37 53.34,39.37 53.98,38.73 53.98,32.38 54.61,31.75 v55.24,31.75 | v61.58,31.75 78.74,31.75 79.38,32.38 79.38,48.26 83.19,52.07 87.63,52.07 88.27,51.44 | 88.27,47.62 88.27,45.41 88.9,44.78 X2.1 | 85.72,60.73 85.72,60.63
  Bottom 1.27: 88.27,47.62 88.27,51.44 88.27,59.99 87.63,60.63 85.72,60.63 | D1.A 85.72,60.73
XTAL1
  Bottom 0.406: 25.4,48.26 22.23,48.26 21.59,48.9 R12.1 21.59,49.66 C1.2 | 25.4,48.26 X1.P$1 | 25.4,48.26 27.3,48.26 27.94,48.9 27.94,49.37 28.57,50 IC1.16

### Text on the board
tNames: 1 | BLK | D11 | EC11E / Encoder | 5V
bNames: Bio4_LCD_v1.1
tValues: Simple spectro / V 1.6.1
bValues: GND | GND | + | GND | GND | GND | GND | GND | + | Simple spectro / V1.6.1
bDocu: N | M | L | K | J | I | H | G | F | E | B | A | C | D | Green | Blue | Red

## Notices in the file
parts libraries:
lpatiny: ©2009 ROFA.cz - modified and updated by Robert Darlington ‹rdarlington@gmail.com›
microbuilder: This work is placed in the public domain, and may be freely used for commercial and non-commercial work with the following conditions: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
